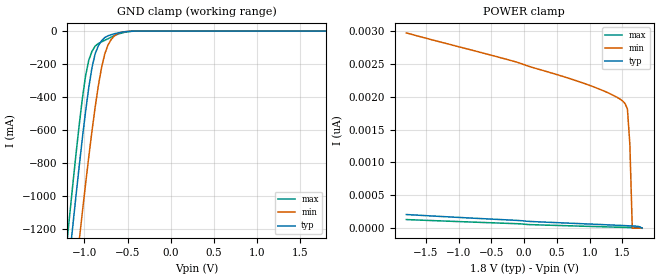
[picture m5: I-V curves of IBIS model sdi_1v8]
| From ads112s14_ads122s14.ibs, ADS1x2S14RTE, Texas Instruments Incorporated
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|   Model sdi_1v8
[Model] sdi_1v8
Model_type Input
Polarity   Non-Inverting
Enable   Active-High
Vinl =  0.540V
Vinh =  1.260V
C_comp   4.000pF   2.000pF   8.000pF
[Model Spec]
Vinh   1.260V   1.155V   1.365V
Vinl   0.540V   0.495V   0.585V
[Temperature Range]   27.000   0.125k   -40.000
[Voltage Range]   1.800V   1.650V   1.980V
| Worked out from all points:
|   GND clamp passes 1 mA (typ) near -0.45 V on its own axis
[GND_clamp]
|Voltage   I(typ)   I(min)   I(max)
-1.8V     -4.499A    -4.387A    -4.584A
-1.208V   -1.559A    -1.997A    -1.316A
-1.171V   -1.369A    -1.813A    -1.122A
-1.134V   -1.183A    -1.63A     -932.1mA
-1.06V    -820.7mA   -1.272A    -571mA
-986mV    -488mA     -927.3mA   -271.8mA
-912mV    -222.4mA   -606.8mA   -123.5mA
-838mV    -88.72mA   -331.1mA   -75.13mA
-764mV    -39.58mA   -139.3mA   -55.93mA
-653mV    -16.25mA   -29.74mA   -27.62mA
-505mV    -2.763mA   -2.319mA   -4.524mA
1.8V      0A         0A         0A
[POWER_clamp]
|Voltage   I(typ)   I(min)   I(max)
-1.8V     207.2pA    2.969nA    130.7pA
-161mV    120.8pA    2.538nA    69.76pA
653mV     77.38pA    2.288nA    36.95pA
1.208V    53.49pA    2.09nA     20.86pA
1.393V    45.32pA    2.004nA    15.58pA
1.504V    40.28pA    1.933nA    12.42pA
1.541V    38.55pA    1.895nA    11.37pA
1.578V    36.8pA     1.81nA     10.32pA
1.615V    35.01pA    1.272nA    9.273pA
1.652V    33.18pA    0A         8.226pA
1.763V    21.8pA     0A         5.09pA
1.8V      0A         0A         4.045pA
